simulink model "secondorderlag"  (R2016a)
settings: Solver=ode45  StartTime=0.0  StopTime=10.0  RelTol=1e-3
model workspace (MAT data in the model file):
  MCOS : class17 (value not decoded)
  tpb2edd403_23e6_44c0_9bbe_931c05806b65 : struct (value not decoded)
undefined symbols (not defined in the file): initialv, initialy, k1, k2, k3, reactiontime, target

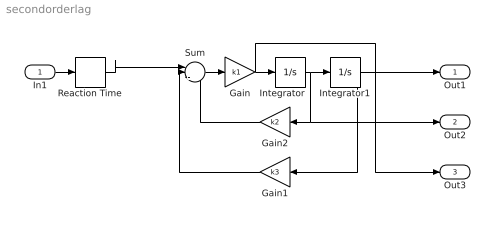
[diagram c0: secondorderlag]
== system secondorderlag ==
  In1 : Inport
  Gain : Gain  Gain=k1
  Gain1 : Gain  Gain=k3
  Gain2 : Gain  Gain=k2
  Integrator : Integrator  InitialCondition=initialv
  Integrator1 : Integrator  InitialCondition=initialy
  Reaction Time : TransportDelay  DelayTime=reactiontime  InitialOutput=target(1)
  Sum : Sum  Inputs=|+--
  Out1 : Outport
  Out2 : Outport  Port=2
  Out3 : Outport  Port=3
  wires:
  Sum/1 -> Gain/1
  Gain1/1 -> Sum/2
  Gain2/1 -> Sum/3
  Integrator1/1 -> Gain1/1, Out1/1
  In1/1 -> Reaction Time/1
  Gain/1 -> Out3/1, Integrator/1
  Integrator/1 -> Gain2/1, Out2/1, Integrator1/1
  Reaction Time/1 -> Sum/1
